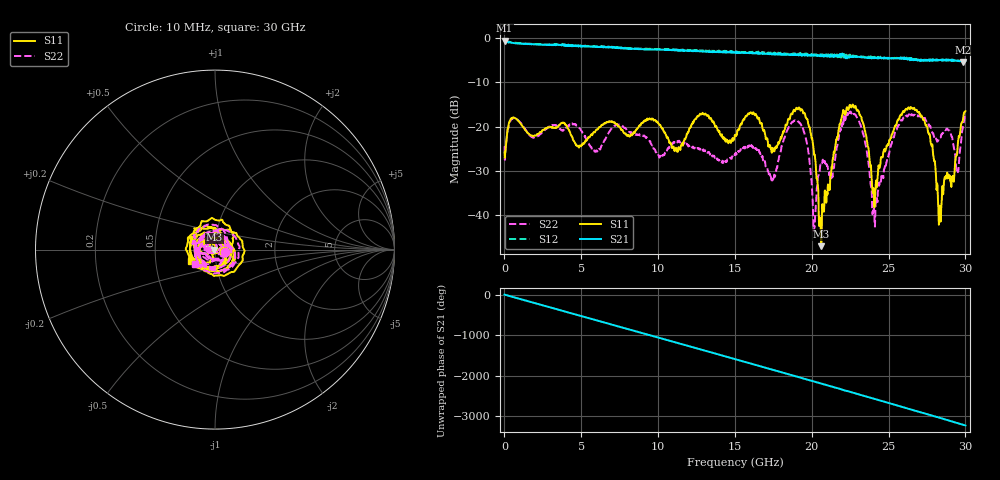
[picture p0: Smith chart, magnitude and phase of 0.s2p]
!Agilent Technologies,E8364B,US42250130,A.04.87.01
!Agilent E8364B: A.04.87.01
!Date: Monday, February 07, 2022 23:44:55
!Correction: S11(Full 2 Port SOLT,1,2) S21(Full 2 Port SOLT,1,2) S12(Full 2 Port SOLT,1,2) S22(Full 2 Port SOLT,1,2)
!S2P File: Measurements: S11, S21, S12, S22:
# Hz S  dB  R 50
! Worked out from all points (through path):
!   1601 points, 10 MHz to 30 GHz, reference 50 ohm
!   highest |S21| = -0.56 dB at 10 MHz (marker M1); lowest = -5.4 dB at 29.87 GHz (marker M2)
!   group delay of S21, straight-line fit = 298 ps
!   lowest |S11| = -47.1 dB at 20.63 GHz (marker M3), VSWR 1.01, Z = 49.6 - j0.0796 ohm
!   |S11| at or under -10 dB: start of sweep to end of sweep
!   |S22| runs from -43.7 to -16.6 dB; largest |S21 - S12| = 0.088
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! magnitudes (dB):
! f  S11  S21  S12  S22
! 10 MHz  -25.9  -0.6  -0.6  -24.5
! 572.3 MHz  -18.0  -1.1  -1.0  -18.1
! 5.015 GHz  -24.3  -1.7  -1.7  -21.0
! 10.02 GHz  -19.3  -2.5  -2.4  -26.5
! 15.01 GHz  -21.9  -3.2  -3.2  -26.4
! 16.13 GHz  -17.0  -3.3  -3.0  -24.6
! 17.48 GHz  -25.4  -3.7  -3.2  -31.8
! 19.05 GHz  -16.0  -3.7  -3.5  -18.6
! 19.65 GHz  -18.2  -3.8  -3.5  -23.3
! 20.01 GHz  -22.6  -3.8  -3.6  -33.5
! 20.22 GHz  -27.2  -3.9  -3.6  -40.6
! 20.63 GHz  -47.1  -4.0  -3.7  -28.4
! 21.3 GHz  -29.3  -4.0  -3.8  -32.0
! 22.17 GHz  -17.3  -4.3  -3.8  -17.7
! 23.23 GHz  -17.9  -4.2  -4.1  -20.3
! 24.08 GHz  -38.3  -4.5  -4.2  -40.7
! 25.01 GHz  -23.8  -4.6  -4.5  -26.2
! 27.06 GHz  -17.2  -5.0  -4.8  -17.7
! 28.35 GHz  -38.6  -4.9  -4.9  -22.6
! 29.49 GHz  -24.5  -5.1  -5.0  -30.0
! 29.87 GHz  -17.8  -5.4  -4.9  -19.8
! 30 GHz  -16.5  -5.2  -5.3  -17.1
